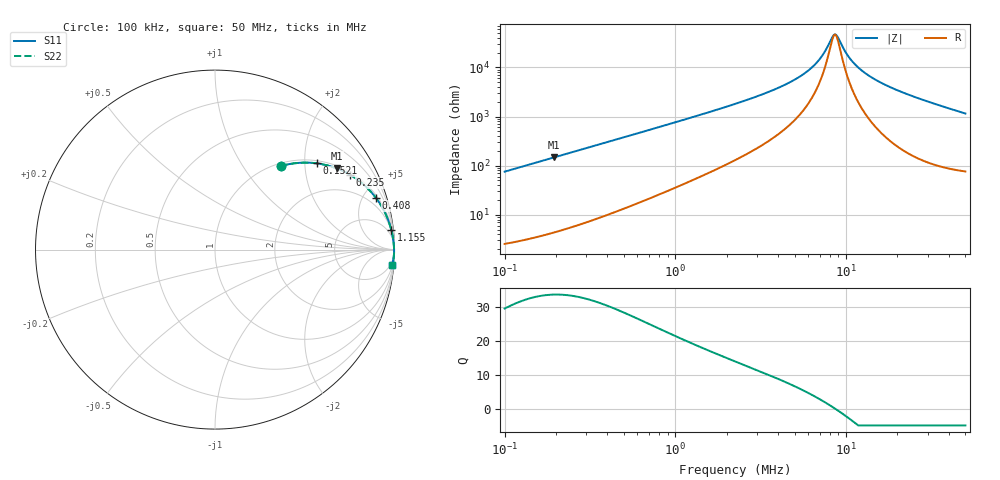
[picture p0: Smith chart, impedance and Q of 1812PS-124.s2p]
# MHz S MA R 50
!Freq  MagS11  AngS11  MagS21  AngS21  MagS12  AngS12  MagS22  AngS22
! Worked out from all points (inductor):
!   801 points, 100 kHz to 50 MHz, reference 50 ohm
!   read as one part in series: L = 120 uH near 103.2 kHz
!   highest Q = 33.7 at 195 kHz (marker M1), where L = 120 uH
!   self-resonance near 8.573 MHz
!   S11 on the Smith chart (normalised r, x): 100 kHz: 1.05, +1.51; 152.1 kHz: 1.07, +2.29; 235 kHz: 1.11, +3.55; 408 kHz: 1.20, +6.16; 1.155 MHz: 2, +18; 50 MHz: 3, -23
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0.1  0.5927 51.7  0.7856 -36.3  0.7856 -36.3  0.5927 51.7
0.152118  0.7428 40.3  0.6474 -47.9  0.6474 -47.9  0.7428 40.3
0.195047  0.8159 33.7  0.5545 -54.6  0.5545 -54.6  0.8159 33.7
0.2350219  0.8601 29.0  0.485 -59.3  0.485 -59.3  0.8601 29.0
0.2831897  0.8953 24.8  0.4189 -63.5  0.4189 -63.5  0.8953 24.8
0.4079829  0.9421 17.8  0.3056 -70.3  0.3056 -70.3  0.9421 17.8
0.7957584  0.98 9.3  0.162 -78.3  0.162 -78.3  0.98 9.3
1.155366  0.9882 6.4  0.1115 -80.7  0.1115 -80.7  0.9882 6.4
2.236068  0.9945 3.2  0.05514 -82.7  0.05514 -82.7  0.9945 3.2
4.327634  0.9969 1.3  0.023 -81.6  0.023 -81.6  0.9969 1.3
5.379161  0.9973 0.9  0.0152 -79.4  0.0152 -79.4  0.9973 0.9
6.332315  0.9976 0.5  0.009877 -75.4  0.009877 -75.4  0.9976 0.5
7.170375  0.9977 0.3  0.006087 -67.7  0.006087 -67.7  0.9977 0.3
8.310792  0.9978 0.1  0.00241 -26.4  0.00241 -26.4  0.9978 0.1
8.639945  0.9979 -0.0  0.002132 3.2  0.002132 3.2  0.9979 -0.0
8.982134  0.9979 -0.1  0.002479 31.9  0.002479 31.9  0.9979 -0.1
10.33014  0.998 -0.3  0.005996 70.0  0.005996 70.0  0.998 -0.3
11.60679  0.998 -0.5  0.009541 77.5  0.009541 77.5  0.998 -0.5
13.87738  0.9979 -0.9  0.01538 81.9  0.01538 81.9  0.9979 -0.9
17.7937  0.9977 -1.4  0.02442 83.9  0.02442 83.9  0.9977 -1.4
27.49123  0.9964 -2.5  0.04428 84.1  0.04428 84.1  0.9964 -2.5
50  0.9906 -4.9  0.08599 81.3  0.08599 81.3  0.9906 -4.9
